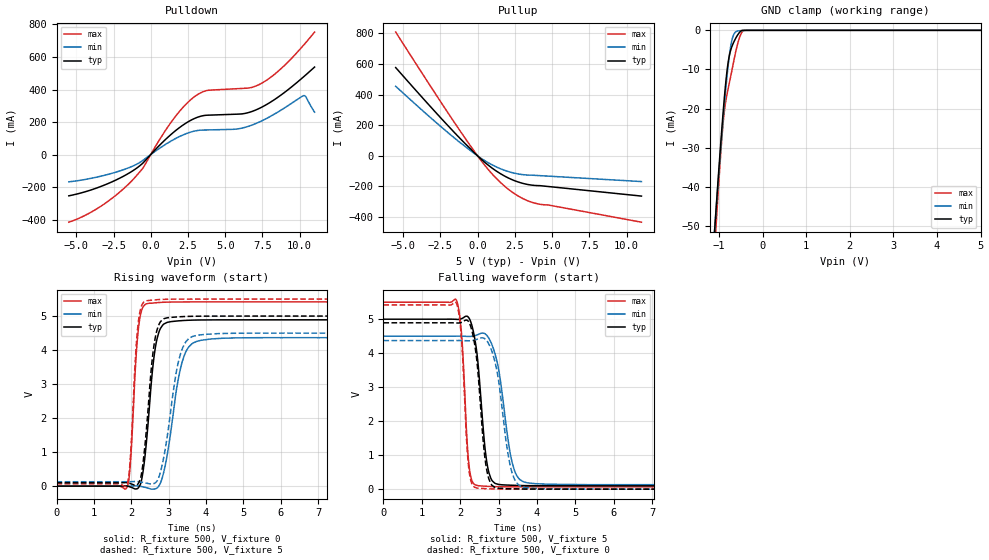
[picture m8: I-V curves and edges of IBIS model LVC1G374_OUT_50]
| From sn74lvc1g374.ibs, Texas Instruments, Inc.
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[Model]   LVC1G374_OUT_50
Model_type  3-state
Enable   Active-Low
Vref =   0
Rref =   500
Cref =   50p
Vmeas =   2.5
| variable   typ   min   max
C_comp   4.99pF   4.17pF   6.36pF
| C_pullup   7.94pF   4.95pF   9.64pF
| C_pulldown   7.39pF   5.76pF   10.46pF
| C_tri-state   4.99pF   4.17pF   6.36pF
[Temperature Range]   40   100   -40
| Ambient temperature   25   85   -40
[Voltage range]   5   4.5   5.5
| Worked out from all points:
|   slope of the pulldown table from 0 to 0.75 V, typ, clamps not added: 10.5 ohm
|   slope of the pullup table from 0 to 0.75 V, typ, clamps not added: 11.8 ohm
|   GND clamp passes 1 mA (typ) near -0.56 V on its own axis
|   rising waveform, R_fixture 500, V_fixture 0: 20-80 % time 246ps typ, 370ps min, 165ps max; typ from 0 V to 4.89 V
|   falling waveform, R_fixture 500, V_fixture 5: 20-80 % time 226ps typ, 327ps min, 149ps max; typ from 5 V to 0.098 V
|   rising waveform, R_fixture 500, V_fixture 5: 20-80 % time 238ps typ, 361ps min, 159ps max; typ from 0.098 V to 5 V
|   falling waveform, R_fixture 500, V_fixture 0: 20-80 % time 219ps typ, 318ps min, 147ps max; typ from 4.89 V to 0 V
[GND Clamp]
| LVC1G374_OUT_50
|   Voltage   I(typ)   I(min)   I(max)
-5.5V     -897.8mA   -832.4mA   -1.016A
-1.115V   -53.65mA   -53.2mA    -58.9mA
-1.08V    -47.86mA   -47.85mA   -52.38mA
-1.05V    -42.97mA   -43.33mA   -46.9mA
-915mV    -22.35mA   -24.01mA   -24.95mA
-870mV    -16.36mA   -18.13mA   -20.06mA
-810mV    -9.836mA   -11.06mA   -16.02mA
-710mV    -4.33mA    -2.831mA   -10.59mA
-595mV    -1.595mA   -242.2uA   -4.449mA
-505mV    -252.5uA   -82.42uA   -1.167mA
-430mV    -5.556uA   -35.43uA   -28.28uA
5V        28.94pA    122nA      715.4pA
[Pulldown]
| LVC1G374_OUT_50
|   Voltage   I(typ)   I(min)   I(max)
-5.5V     -253.9mA   -167.9mA   -416mA
-3.405V   -198.2mA   -134.3mA   -321.3mA
-1.385V   -110.1mA   -77.76mA   -172.1mA
-505mV    -50.36mA   -34.24mA   -80.09mA
1.515V    135.7mA    90.96mA    217.2mA
2.88V     219.5mA    143.2mA    352mA
3.795V    242.1mA    151.3mA    394.3mA
5.85V     248.6mA    158mA      405.4mA
7.4V      289mA      204.9mA    436.3mA
8.705V    363.4mA    271mA      524.8mA
10.28V    479.6mA    362.7mA    674.8mA
11V       538.2mA    260.8mA    753.3mA
[Pullup]
| LVC1G374_OUT_50
|   Voltage   I(typ)   I(min)   I(max)
-5.5V     577mA      454.6mA    809mA
-2.245V   224mA      172.9mA    318.8mA
-15mV     1.399mA    1.048mA    2.031mA
515mV     -44.85mA   -33.24mA   -65.78mA
1.045V    -84.88mA   -62.15mA   -125.6mA
1.575V    -118.7mA   -85.68mA   -177.4mA
2.1V      -146.1mA   -103.7mA   -220.9mA
3.005V    -178.9mA   -122.3mA   -277.5mA
3.91V     -193.7mA   -127.7mA   -310.7mA
4.725V    -200mA     -132.3mA   -320.7mA
11V       -262.8mA   -168mA     -433.4mA
[Ramp]
| LVC1G374_OUT_50
| variable   typ   min   max
dV/dt_r   2.98/2.55E-10   2.67/3.87E-10   3.30/1.72E-10
dV/dt_f   2.99/2.36E-10   2.68/3.45E-10   3.31/1.54E-10
R_load = 500
[Rising Waveform]
| LVC1G374_OUT_50
R_fixture =   500
C_fixture =   0
L_fixture =   0
V_fixture =   0
V_fixture_min = 0
V_fixture_max = 0
|   Time   V(typ)   V(min)   V(max)
0s        198.4pV    4.048nV    1.782nV
1.88ns    4.405mV    -281.9uV   -50.38mV
1.975ns   -24.65mV   735.7uV    633mV
2.195ns   -43.5mV    3.128mV    4.649V
2.46ns    1.948V     -61.99mV   5.374V
2.615ns   3.836V     -85.13mV   5.386V
2.78ns    4.63V      87.05mV    5.402V
3.365ns   4.867V     3.652V     5.415V
3.87ns    4.885V     4.288V     5.417V
24.99ns   4.89V      4.367V     5.417V
[Falling Waveform]
| LVC1G374_OUT_50
R_fixture =   500
C_fixture =   0
L_fixture =   0
V_fixture =   5
V_fixture_min = 4.5
V_fixture_max = 5.5
|   Time   V(typ)   V(min)   V(max)
0s        5V         4.5V       5.5V
1.905ns   4.995V     4.5V       5.553V
2.035ns   5.016V     4.5V       4.572V
2.235ns   5.022V     4.492V     649.1mV
2.465ns   3.686V     4.549V     103.2mV
2.65ns    1.165V     4.567V     87.16mV
2.795ns   327.1mV    4.333V     78.99mV
3.36ns    114.4mV    752.2mV    69.57mV
3.75ns    103.9mV    186.3mV    68.31mV
24.99ns   98.28mV    129.8mV    67.62mV
[Rising Waveform]
| LVC1G374_OUT_50
R_fixture =   500
C_fixture =   0
L_fixture =   0
V_fixture =   5
V_fixture_min = 4.5
V_fixture_max = 5.5
|   Time   V(typ)   V(min)   V(max)
0s        98.26mV    129.8mV    67.61mV
1.88ns    102.5mV    129.5mV    32.88mV
1.97ns    76.25mV    130.4mV    725.4mV
2.18ns    61.62mV    134.5mV    4.722V
2.415ns   1.771V     86.93mV    5.451V
2.585ns   3.939V     69.05mV    5.471V
2.75ns    4.768V     294.8mV    5.485V
3.295ns   4.979V     3.788V     5.498V
3.76ns    4.996V     4.434V     5.5V
24.99ns   5V         4.5V       5.5V
[Falling Waveform]
| LVC1G374_OUT_50
R_fixture =   500
C_fixture =   0
L_fixture =   0
V_fixture =   0
V_fixture_min = 0
V_fixture_max = 0
|   Time   V(typ)   V(min)   V(max)
0s        4.893V     4.372V     5.419V
1.9ns     4.889V     4.372V     5.473V
2.035ns   4.909V     4.372V     4.413V
2.22ns    4.923V     4.365V     644.2mV
2.43ns    3.817V     4.404V     34.27mV
2.62ns    1.165V     4.439V     17.67mV
2.75ns    288.8mV    4.258V     10.97mV
3.325ns   12.94mV    585.8mV    1.77mV
3.72ns    4.384mV    42.4mV     624.6uV
24.99ns   11.04uV    18.07uV    7.677uV
